(* This function block represents one IEC 60870-5-101 master->slave connection channel *)
FUNCTION_BLOCK FB_IEC870_5_101M
VAR_IN_OUT
	hSerial		: T_HSERIALCTRL;(* Serial connection control handle *)
	stProcData	: ST_IEC870_5_101MProcData;(* Process data send to or received from IEC 60870-5-101 slave device *)
	fbLog		: FB_IEC870_DebugLogFifo;(* Simple log buffer. We store/log here all our received slave data and other messages *)
END_VAR
VAR_INPUT
	protPara	: ST_IEC870_5_101ProtocolParams := ( eType := eIEC870_101_MASTER );(* Serial link transport protocol parameters *)
	sysPara		: ST_IEC870_5_101MSysPara;(* System parameter *)
	bEnable		: BOOL := TRUE; (* Enables/disables communication channel *)
END_VAR
VAR
	fbProtocol	: FB_IEC870_5_101TProtocol;(* IEC60870-5-101 transport *)
	fbServices	: FB_IEC870_5_101MServices;(* IEC60870-5-101 master services *)
	fbClock		: FB_LocalSystemTime;(* Internal clock: Local windows system time *)
	buffer		: ST_IEC870_5_101TBuffer;(* TX/RX data buffer *)
	nState		: BYTE;
	bReset 		: BOOL;(* Rising edge at this input resets service execution *)
END_VAR

fbClock( bEnable := TRUE, dwCycle := 1 );(* Get local Windows System Time *)
IF NOT fbClock.bValid THEN
	RETURN;
END_IF

CASE nState OF
	0:	(* Init step *)
		IF bEnable THEN
			fbLog( sPrefix := CONCAT( 'IEC 60870-5-101M, linkAddr:', CONCAT( DWORD_TO_STRING( protPara.linkAddr ), CONCAT( ', CAA:', DWORD_TO_STRING( sysPara.asduAddr ) ) ) ) );
		
			(* Initialize the max. asdu size, frame format params and buffer debug mode *)
			buffer.eDbg 	:= sysPara.eDbgAsdu;(* Enable/disable debug output of asdu data *)
			buffer.asduSize	:= F_iecApdu101ToAsduLen( protPara.FRAMELength, protPara.eLinkAddrSize );(* Configure the max. asdu frame length *)
			buffer.asduFmt	:= sysPara.asduFmt;(* Set the frame format parameters (octet sizes) *)

			bReset			:= TRUE;
			
			(* Reset protocol function block and restart data transfer *)
			fbProtocol.INIT( hSerial := hSerial, buffer	:= buffer, protPara := protPara, bOutDbg := sysPara.bDbgLink );
			nState := 1;
		END_IF

	1: (* Establish connection and exchange data *)
		IF bEnable THEN
			fbProtocol( hSerial := hSerial, buffer := buffer );
			IF NOT fbProtocol.bError THEN
				IF fbProtocol.eState = eSERIALLINK_ESTABLISHED THEN

					(* Link established => exchange data *)
					fbServices( buffer := buffer, sysPara := sysPara, bReset := bReset, stProcData := stProcData, fbClock := fbClock, fbLog := fbLog );

				END_IF
			ELSE (* Error => Reset connection *)
				fbLog.A_LogError( sPut := CONCAT( '::Transport interface error: 0x', DWORD_TO_HEXSTR( fbProtocol.nErrID, 8, FALSE ) ) );
				nState := 0;
			END_IF
		ELSE (* Stop communication *)
			nState := 0;
		END_IF

END_CASE

END_FUNCTION_BLOCK
